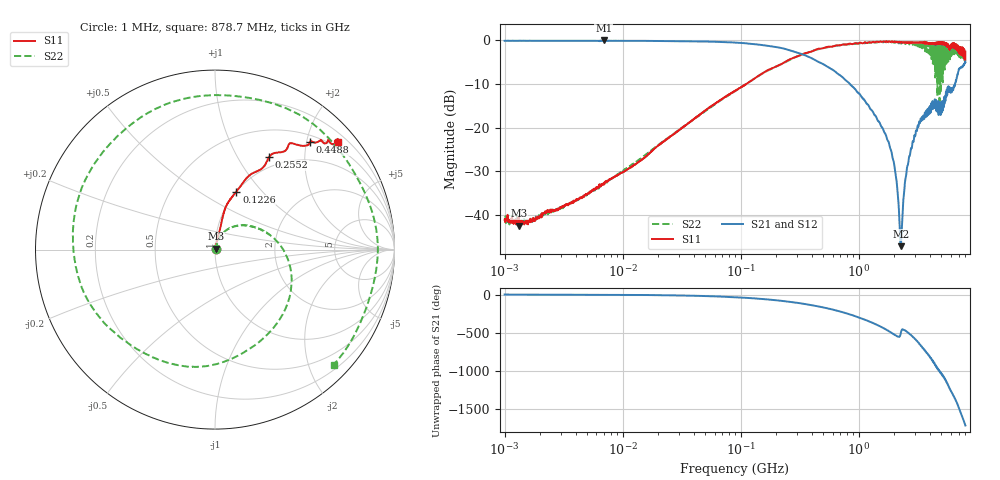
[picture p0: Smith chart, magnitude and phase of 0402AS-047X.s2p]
!s-Parameter Generated by FASTRON Sdn. Bhd.
!FASTRON P/N : 0402AS-047X
!Keysight Technologies: E5071C_MY46733604_B.14.02
!Date: Mon Dec 01 10:47:08 2025
!Version  :Rev00  Mon Dec 01 10:47:08 2025
!Data & Calibration Information:
!Freq  S11:SOLT2(ON)  S21:SOLT2(ON)  S12:SOLT2(ON)  S22:SOLT2(ON)
!PortZ  Port1:50+j0  Port2:50+j0
!When reading reference impedance value at option line is always used.
! Remarks : This data is being provided solely for informational purposes.
# Hz S dB R 50
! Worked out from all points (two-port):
!   1601 points, 1 MHz to 8 GHz, reference 50 ohm
!   highest |S21| = 0.00 dB at 6.912 MHz (marker M1); lowest = -47.2 dB at 2.267 GHz (marker M2)
!   |S21| within 3 dB of the highest: start of sweep to 317.7 MHz
!   lowest |S11| = -42.5 dB at 1.323 MHz (marker M3), VSWR 1.02, Z = 50.6 + j0.447 ohm
!   |S11| at or under -10 dB: start of sweep to 111.3 MHz
!   |S22| runs from -42.2 to -0.2 dB; largest |S21 - S12| = 0.023
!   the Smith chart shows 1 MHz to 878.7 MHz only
!   S11 on the Smith chart (normalised r, x): 1 MHz: 1.02, +0.01; 122.6 MHz: 1.00, +0.73; 255.2 MHz: 0.85, +1.37; 448.8 MHz: 0.62, +2.07; 878.7 MHz: 0.39, +2.62
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1000000  -41.20 28.6  -0.08 -0.4  -0.07 -0.5  -41.10 23.5
1323440  -42.50 36.1  -0.08 -0.6  -0.07 -0.5  -41.90 25.6
4479405  -36.00 62.4  -0.08 -1.9  -0.07 -1.9  -36.10 61.9
6911657  -33.10 64.8  0.00 -3.3  -0.16 -2.9  -32.80 63.1
2.00676e7  -24.10 76.0  -0.11 -8.2  -0.11 -8.2  -24.00 70.4
8.994653e7  -11.50 74.8  -0.49 -35.5  -0.48 -35.5  -11.60 27.0
1.226011e8  -9.25 69.8  -0.76 -47.8  -0.75 -47.8  -9.23 8.3
2.552003e8  -4.45 59.7  -2.19 -94.5  -2.18 -94.5  -4.57 -72.7
4.006501e8  -2.51 50.7  -4.09 -141.0  -4.08 -141.0  -2.42 -155.0
4.488364e8  -1.94 48.4  -4.83 -155.0  -4.81 -155.0  -2.06 -180.0
6.42063e8  -1.11 44.2  -7.31 151.0  -7.30 151.0  -1.23 75.8
8.787371e8  -0.84 41.1  -10.50 89.7  -10.50 89.5  -0.72 -44.1
1.131415e9  -0.42 44.7  -13.90 27.8  -13.90 27.7  -0.62 -173.0
1.334081e9  -0.32 49.8  -16.70 -18.3  -16.70 -18.4  -0.49 88.4
1.542898e9  -0.29 56.0  -19.60 -64.2  -19.60 -64.3  -0.32 -10.3
1.7949e9  -0.22 62.6  -23.40 -121.0  -23.40 -121.0  -0.43 -132.0
2.061212e9  -0.40 68.6  -31.00 -177.0  -31.00 -177.0  -0.35 99.9
2.266813e9  -0.47 72.0  -47.20 -147.0  -47.20 -147.0  -0.56 -2.9
2.618947e9  -0.49 81.1  -28.20 -141.0  -28.20 -141.0  -0.42 -175.0
2.985754e9  -0.44 91.4  -21.90 137.0  -21.90 137.0  -0.88 3.5
3.345355e9  -0.50 100.0  -17.90 51.3  -17.90 50.7  -1.46 -172.0
8e9  -2.55 -115.0  -5.00 81.8  -5.05 81.6  -4.68 118.0
